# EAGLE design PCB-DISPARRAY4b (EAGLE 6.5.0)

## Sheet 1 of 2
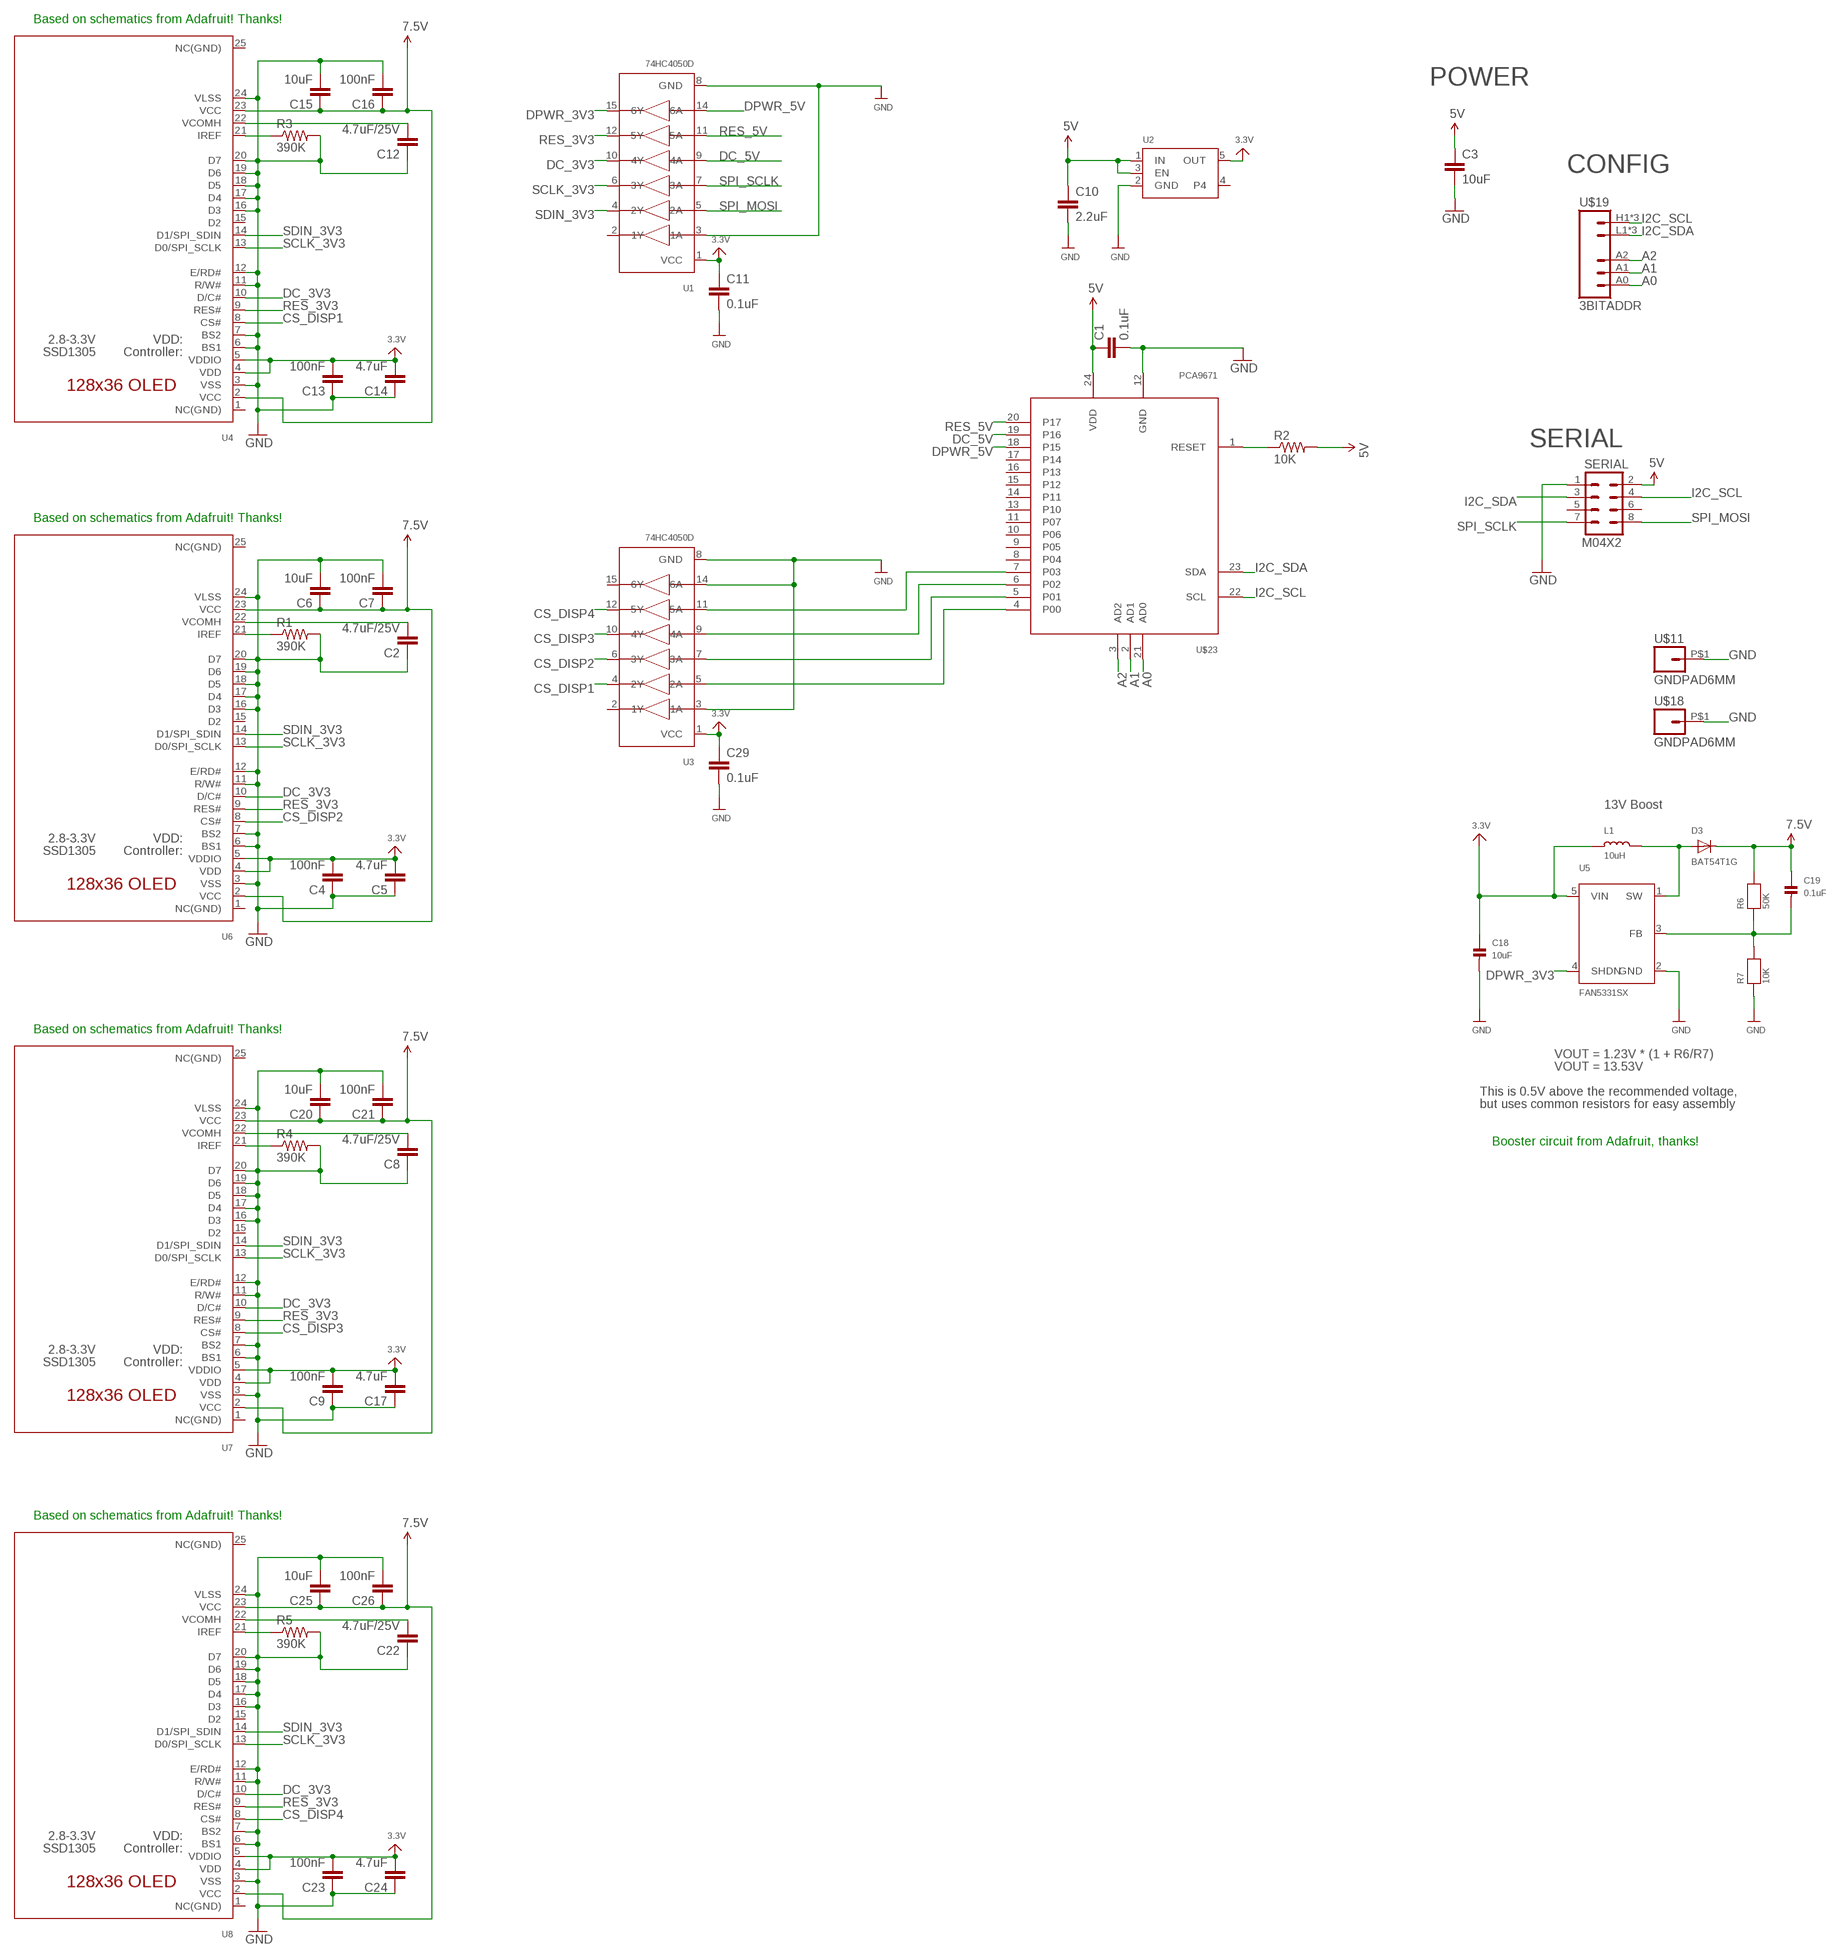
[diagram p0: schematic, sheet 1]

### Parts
C1  0.1uF  CAP0603-CAP  [0603-CAP]
C2  4.7uF/25V  CAP0805  [0805]
C3  10uF  CAP0805  [0805]
C4  100nF  CAP0603-CAP  [0603-CAP]
C5  4.7uF  CAP0603-CAP  [0603-CAP]
C6  10uF  CAP0805  [0805]
C7  100nF  CAP0603-CAP  [0603-CAP]
C8  4.7uF/25V  CAP0805  [0805]
C9  100nF  CAP0603-CAP  [0603-CAP]
C10  2.2uF  CAP0603-CAP  [0603-CAP]
C11  0.1uF  CAP0603-CAP  [0603-CAP]
C12  4.7uF/25V  CAP0805  [0805]
C13  100nF  CAP0603-CAP  [0603-CAP]
C14  4.7uF  CAP0603-CAP  [0603-CAP]
C15  10uF  CAP0805  [0805]
C16  100nF  CAP0603-CAP  [0603-CAP]
C17  4.7uF  CAP0603-CAP  [0603-CAP]
C18  10uF  CAP_CERAMIC0805  [0805]
C19  0.1uF  CAP_CERAMIC0603  [0603]
C20  10uF  CAP0805  [0805]
C21  100nF  CAP0603-CAP  [0603-CAP]
C22  4.7uF/25V  CAP0805  [0805]
C23  100nF  CAP0603-CAP  [0603-CAP]
C24  4.7uF  CAP0603-CAP  [0603-CAP]
C25  10uF  CAP0805  [0805]
C26  100nF  CAP0603-CAP  [0603-CAP]
C29  0.1uF  CAP0603-CAP  [0603-CAP]
D3  BAT54T1G  DIODESOD-123  [SOD-123]
L1  10uH  INDUCTOR  [INDUCTOR_1007]
R1  390K  RESISTOR0603-RES  [0603-RES]
R2  10K  RESISTOR0603-RES  [0603-RES]
R3  390K  RESISTOR0603-RES  [0603-RES]
R4  390K  RESISTOR0603-RES  [0603-RES]
R5  390K  RESISTOR0603-RES  [0603-RES]
R6  50K  RESISTOR0603  [0603]
R7  10K  RESISTOR0603  [0603]
SERIAL  M04X2  [2X4]
U1  74HC4050D  74HC4050DTSSOP16  [TSSOP16]
U2  VREG_SOT23-5  [SOT23-5]
U3  74HC4050D  74HC4050DTSSOP16  [TSSOP16]
U4  ER-OLED011-1TOP  [ER-OLED011-1]
U5  FAN5331SX  FAN5331  [SOT23-5]
U6  ER-OLED011-1TOP  [ER-OLED011-1]
U7  ER-OLED011-1TOP  [ER-OLED011-1]
U8  ER-OLED011-1TOP  [ER-OLED011-1]
U$11  GNDPAD6MM  [3.2MMPAD6MM]
U$18  GNDPAD6MM  [3.2MMPAD6MM]
U$19  3BITADDR  [3BITADDR]
U$23  PCA9671  [TSSOP24]

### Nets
3.3V [Power]: C4.2 C5.2 C9.2 C11.1 C13.2 C14.2 C17.2 C18.1 C23.2 C24.2 C29.1 L1.P$1 U1.1(VCC) U2.5(OUT) U3.1(VCC) U4.4(VDD) U4.5(VDDIO) U5.5(VIN) U6.4(VDD) U6.5(VDDIO) U7.4(VDD) U7.5(VDDIO) U8.4(VDD) U8.5(VDDIO)
5V [Power]: C1.1 C3.1 C10.1 R2.2 SERIAL.2 U2.1(IN) U2.3(EN) U$23.24(VDD)
7.5V [Power]: C6.1 C7.1 C15.1 C16.1 C19.1 C20.1 C21.1 C25.1 C26.1 D3.C R6.2 U4.2(VCC) U4.23(VCC) U6.2(VCC) U6.23(VCC) U7.2(VCC) U7.23(VCC) U8.2(VCC) U8.23(VCC)
A0: U$19.A0 U$23.21(AD0)
A1: U$19.A1 U$23.2(AD1)
A2: U$19.A2 U$23.3(AD2)
CS_DISP1: U3.4(2Y) U4.8(CS#)
CS_DISP2: U3.6(3Y) U6.8(CS#)
CS_DISP3: U3.10(4Y) U7.8(CS#)
CS_DISP4: U3.12(5Y) U8.8(CS#)
DC_3V3: U1.10(4Y) U4.10(D/C#) U6.10(D/C#) U7.10(D/C#) U8.10(D/C#)
DC_5V: U1.9(4A) U$23.19(P16)
DPWR_3V3: U1.15(6Y) U5.4(SHDN)
DPWR_5V [Power]: U1.14(6A) U$23.18(P15)
GND [Power]: C1.2 C2.1 C3.2 C4.1 C5.1 C6.2 C7.2 C8.1 C9.1 C10.2 C11.2 C12.1 C13.1 C14.1 C15.2 C16.2 C17.1 C18.2 C20.2 C21.2 C22.1 C23.1 C24.1 C25.2 C26.2 C29.2 R1.2 R3.2 R4.2 R5.2 R7.1 SERIAL.1 U1.3(1A) U1.8(GND) U2.2(GND) U3.3(1A) U3.8(GND) U3.14(6A) U4.3(VSS) U4.6(BS1) U4.7(BS2) U4.11(R/W#) U4.12(E/RD#) U4.16(D3) U4.17(D4) U4.18(D5) U4.19(D6) U4.20(D7) U4.24(VLSS) U5.2(GND) U6.3(VSS) U6.6(BS1) U6.7(BS2) U6.11(R/W#) U6.12(E/RD#) U6.16(D3) U6.17(D4) U6.18(D5) U6.19(D6) U6.20(D7) U6.24(VLSS) U7.3(VSS) U7.6(BS1) U7.7(BS2) U7.11(R/W#) U7.12(E/RD#) U7.16(D3) U7.17(D4) U7.18(D5) U7.19(D6) U7.20(D7) U7.24(VLSS) U8.3(VSS) U8.6(BS1) U8.7(BS2) U8.11(R/W#) U8.12(E/RD#) U8.16(D3) U8.17(D4) U8.18(D5) U8.19(D6) U8.20(D7) U8.24(VLSS) U$11.P$1 U$18.P$1 U$23.12(GND)
I2C_SCL: SERIAL.4 U$19.H1(VCC) U$19.H2(VCC) U$19.H3(VCC) U$23.22(SCL)
I2C_SDA: SERIAL.3 U$19.L1(GND) U$19.L2(GND) U$19.L3(GND) U$23.23(SDA)
N$1: R2.1 U$23.1(RESET)
N$2: R1.1 U6.21(IREF)
N$3: C2.2 U6.22(VCOMH)
N$4: R4.1 U7.21(IREF)
N$5: R3.1 U4.21(IREF)
N$6: C8.2 U7.22(VCOMH)
N$7: R5.1 U8.21(IREF)
N$8: C22.2 U8.22(VCOMH)
N$10: C12.2 U4.22(VCOMH)
N$14 [Power]: D3.A L1.P$2 U5.1(SW)
N$15: C19.2 R6.1 R7.2 U5.3(FB)
N$29: U3.5(2A) U$23.4(P00)
N$30: U3.7(3A) U$23.5(P01)
N$31: U3.9(4A) U$23.6(P02)
N$32: U3.11(5A) U$23.7(P03)
RES_3V3: U1.12(5Y) U4.9(RES#) U6.9(RES#) U7.9(RES#) U8.9(RES#)
RES_5V: U1.11(5A) U$23.20(P17)
SCLK_3V3: U1.6(3Y) U4.13(D0/SPI_SCLK) U6.13(D0/SPI_SCLK) U7.13(D0/SPI_SCLK) U8.13(D0/SPI_SCLK)
SDIN_3V3: U1.4(2Y) U4.14(D1/SPI_SDIN) U6.14(D1/SPI_SDIN) U7.14(D1/SPI_SDIN) U8.14(D1/SPI_SDIN)
SPI_MOSI: SERIAL.8 U1.5(2A)
SPI_SCLK: SERIAL.7 U1.7(3A)
Unconnected: SERIAL.5 SERIAL.6 U1.2(1Y) U2.4 U3.2(1Y) U3.15(6Y) U4.1(NC(GND)) U4.15(D2) U4.25(NC(GND)) U6.1(NC(GND)) U6.15(D2) U6.25(NC(GND)) U7.1(NC(GND)) U7.15(D2) U7.25(NC(GND)) U8.1(NC(GND)) U8.15(D2) U8.25(NC(GND)) U$23.8(P04) U$23.9(P05) U$23.10(P06) U$23.11(P07) U$23.13(P10) U$23.14(P11) U$23.15(P12) U$23.16(P13) U$23.17(P14)

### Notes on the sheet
- Based on schematics from Adafruit! Thanks!
- POWER
- CONFIG
- SERIAL
- Based on schematics from Adafruit! Thanks!
- 13V Boost
- Based on schematics from Adafruit! Thanks!
- VOUT = 1.23V * (1 + R6/R7)
- VOUT = 13.53V
- This is 0.5V above the recommended voltage,
- but uses common resistors for easy assembly
- Booster circuit from Adafruit, thanks!
- Based on schematics from Adafruit! Thanks!

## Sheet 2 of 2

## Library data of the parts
C1-C17 C20-C26 C29 = SparkFun:CAP: Capacitor
C18 C19 = microbuilder:CAP_CERAMIC: Ceramic Capacitors
D3 = microbuilder:DIODE: Diode
L1 = microbuilder:INDUCTOR: Inductors
R1-R5 = SparkFun:RESISTOR: Resistor
R6 R7 = microbuilder:RESISTOR: Resistors
SERIAL = SparkFun:M04X2
U1 U3 = SKAARHOJ:74HC4050D: 6-channel level shifter 74HC4050D - 2V-6V Supply Digikey: 74HC4050D,653-ND Mouser: 771-74HC4050D-T
U2 = microbuilder:VREG_SOT23-5: SOT23-5 Fixed Voltage Regulators To better organise some of the SOT23-5 fixed voltage regulators in this library, this new part was created. Part Current Out V Out V In V Dropout Digikey Part No. ADP121 150mA 3.3V 3.4-5.5V 0.09V @ 150mA ADP121-AUJZ33R7CT-ND ADP121 150mA 3.0V 3.1-5.5V 0.09V @ 150mA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
U4 U6-U8 = SKAARHOJ:ER-OLED011-1: UG-2864HSWEG01 OLED display Both 1.3" and 0.96" models share the same FPC tab footprint, only the screen dimensions vary.
U5 = microbuilder:FAN5331: FAN5331 - LED/OLED 20V Boost Converter Digikey: FAN5331SXCT-ND
U$11 U$18 = SKAARHOJ:GNDPAD
U$19 = SKAARHOJ:3BITADDR
U$23 = SKAARHOJ:PCA9671

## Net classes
0 default: width 0.203 mm, drill 0.305 mm, clearance 0.203 mm
1 Power: width 0.305 mm, drill 0.406 mm, clearance 0.203 mm

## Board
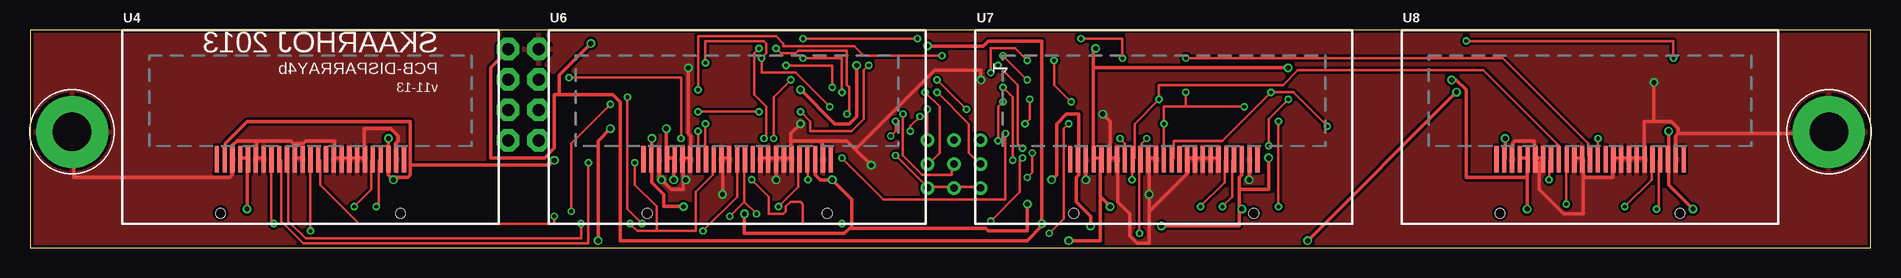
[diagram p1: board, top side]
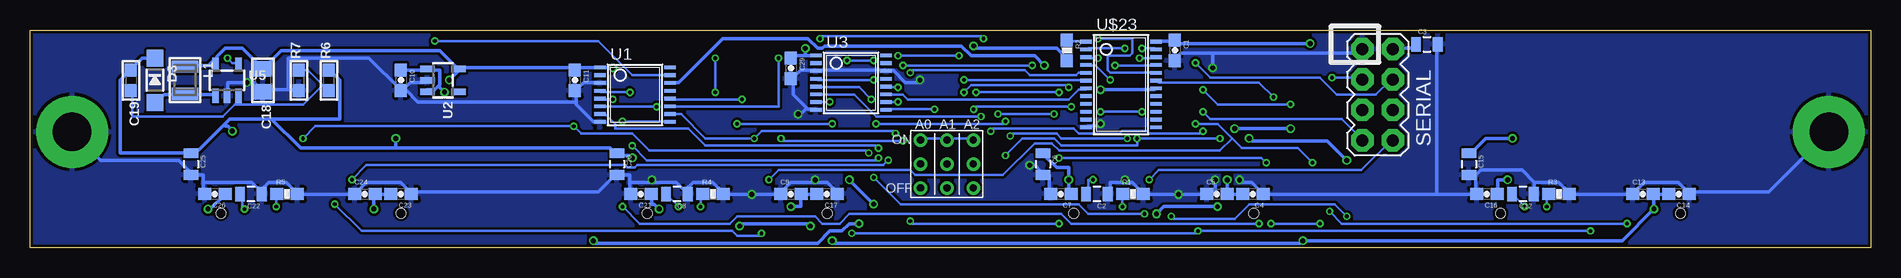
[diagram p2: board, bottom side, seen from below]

Size 153.42 x 18.2 mm. Coordinates in mm from the lower left corner, seen from the top.
Outline: 153.42,0 153.42,18.2 0,18.2 0,0 153.42,0
Copper layers (1*16): Top 0.035mm / dielectric 1.5mm / Bottom 0.035mm
Design rules "Fusion_eagle_rule_v1.1": minimum track width 6mil, minimum drill 12mil, track to track 6mil, track to pad 6mil, pad to pad 6mil, via to via 6mil, smd to smd 0mil, copper to edge 10mil, drill to drill 10mil, minimum pad ring 10mil, minimum via ring 6mil, stop-mask expansion 2mil, vias tented up to drill 100mil, thermal gap 10mil

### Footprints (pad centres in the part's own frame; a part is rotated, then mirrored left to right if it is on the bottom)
0603-CAP = smd 1.1 x 1: 1 -0.85,0; 2 0.85,0
0805 = smd 0.8 x 1.2: 1 -0.9,0; 2 0.9,0
0805' = smd 1.3 x 1.5: 1 -0.95,0; 2 0.95,0
0603 = smd 1.1 x 1: 1 -0.85,0; 2 0.85,0
SOD-123 = smd 1.4 x 1.4: A 1.85,0; C -1.85,0
INDUCTOR_1007 = smd 1.016 x 2.2: P$1 -1.127,0; P$2 1.127,0
0603-RES = smd 1.1 x 1: 1 -0.85,0; 2 0.85,0
2X4 = drill 1.016 pad 1.88 octagon: 1 -3.81,-1.27; 2 -3.81,1.27; 3 -1.27,-1.27; 4 -1.27,1.27; 5 1.27,-1.27; 6 1.27,1.27; 7 3.81,-1.27; 8 3.81,1.27
TSSOP16 = smd 0.305 x 0.991: 1 -3.575,-2.918; 2 -2.925,-2.918; 3 -2.275,-2.918; 4 -1.625,-2.918; 5 -0.975,-2.918; 6 -0.325,-2.918; 7 0.325,-2.918; 8 0.975,-2.918; 9 0.975,2.918; 10 0.325,2.918; 11 -0.325,2.918; 12 -0.975,2.918; 13 -1.625,2.918; 14 -2.275,2.918; 15 -2.925,2.918; 16 -3.575,2.918
SOT23-5 = smd 0.55 x 1.2: 1 -0.95,-1.3; 2 0,-1.3; 3 0.95,-1.3; 4 0.95,1.3; 5 -0.95,1.3
ER-OLED011-1 = smd 0.35 x 2.2: 1 -7.8,-2.7; 2 -7.15,-2.7; 3 -6.5,-2.7; 4 -5.85,-2.7; 5 -5.2,-2.7; 6 -4.55,-2.7; 7 -3.9,-2.7; 8 -3.25,-2.7; 9 -2.6,-2.7; 10 -1.95,-2.7; 11 -1.3,-2.7; 12 -0.65,-2.7; 13 0,-2.7; 14 0.65,-2.7; 15 1.3,-2.7; 16 1.95,-2.7; 17 2.6,-2.7; 18 3.25,-2.7; 19 3.9,-2.7; 20 4.55,-2.7; 21 5.2,-2.7; 22 5.85,-2.7; 23 6.5,-2.7; 24 7.15,-2.7; 25 7.8,-2.7 | hole 0.8: -7.5,-7.2; 7.5,-7.2
3.2MMPAD6MM = drill 3.2 pad 6: P$1 0,0
3BITADDR = drill 0.6: A0 -2.2,0; A1 0,0; A2 2.2,0; H1 -2.2,2; H2 0,2; H3 2.2,2; L1 -2.2,-2; L2 0,-2; L3 2.2,-2
TSSOP24 = smd 0.305 x 0.991: 1 -4.225,-2.918; 2 -3.575,-2.918; 3 -2.925,-2.918; 4 -2.275,-2.918; 5 -1.625,-2.918; 6 -0.975,-2.918; 7 -0.325,-2.918; 8 0.325,-2.918; 9 0.975,-2.918; 10 1.625,-2.918; 11 2.275,-2.918; 12 2.925,-2.918; 13 2.925,2.918; 14 2.275,2.918; 15 1.625,2.918; 16 0.975,2.918; 17 0.325,2.918; 18 -0.325,2.918; 19 -0.975,2.918; 20 -1.625,2.918; 21 -2.275,2.918; 22 -2.925,2.918; 23 -3.575,2.918; 24 -4.225,2.918

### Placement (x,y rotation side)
C1  58,16.5 270 bottom
C2  64.5,4.5 180 bottom
C3  37,17 0 bottom
C4  51.5,4.5 180 bottom
C5  54.5,4.5 0 bottom
C6  69,7 270 bottom
C7  67.5,4.5 180 bottom
C8  99.5,4.5 180 bottom
C9  90,4.5 0 bottom
C10  122.5,14 270 bottom
C11  108,14 270 bottom
C12  29,4.5 180 bottom
C13  19,4.5 0 bottom
C14  16,4.5 180 bottom
C15  33.5,7 270 bottom
C16  32,4.5 180 bottom
C17  87,4.5 180 bottom
C18  10uF  [0805']  134,14 270 bottom
C19  145,14 270 bottom
C20  104.5,7 270 bottom
C21  102.5,4.5 180 bottom
C22  135,4.5 180 bottom
C23  122.5,4.5 180 bottom
C24  125.5,4.5 0 bottom
C25  140,7 270 bottom
C26  138,4.5 180 bottom
C29  90,15 270 bottom
D3  143,14 270 bottom
L1  140.5,14 270 bottom
R1  61.5,4.5 0 bottom
R2  67,16.5 270 bottom
R3  26,4.5 0 bottom
R4  96.5,4.5 0 bottom
R5  132,4.5 0 bottom
R6  128.5,14 90 bottom
R7  131,14 90 bottom
SERIAL  41.12,12.79 270 bottom
U1  103,11.5 270 bottom
U2  119,14 270 bottom
U3  85,12.5 270 bottom
U4  23.37,10.1 0 top
U5  137,14 0 bottom
U6  58.93,10.1 0 top
U7  94.49,10.1 0 top
U8  130,10.1 0 top
U$11  149.92,9.7 0 top
U$18  3.5,9.7 0 top
U$19  77,7 0 bottom
U$23  62.5,13 270 bottom

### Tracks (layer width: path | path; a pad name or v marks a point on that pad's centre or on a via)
3.3V  (via drill 0.41)
  Top 0.305: v53.65,5.69 53.65,7.32 U6.5 53.65,7.52 53.24,7.52 U6.4 53.03,7.52 v53.03,9.96 | v18.09,3.25 18.09,7.32 U4.5 18.09,7.52 17.68,7.52 U4.4 | v48.36,9.96 47.35,8.94 v47.35,0.61 | 89.31,4.17 89.2,4.27 89.2,7.32 U7.5 89.2,7.52 88.8,7.52 U7.4 88.59,7.52 88.59,15.04 | 89.31,4.17 v90.02,3.45 | v88.8,16.66 88.59,16.46 88.59,15.04 | 124.77,5.89 124.77,7.32 U8.5 124.77,7.52 124.16,7.52 U8.4 | 124.77,5.89 v124.77,3.25 | 124.77,5.89 119.69,5.89 119.69,13.21 118.87,14.02 v118.47,14.02 | v104.85,15.04 88.59,15.04 | v86.56,0.61 89.2,0.61 89.2,4.06 89.31,4.17
  Bottom 0.305: C4.2 52.43,4.47 53.65,4.47 C5.2 53.65,4.67 v53.65,5.69 | 18.09,4.47 16.87,4.47 C14.2 | 18.09,4.47 v18.09,3.25 20.73,0.61 v47.35,0.61 47.55,0.41 86.36,0.41 v86.56,0.61 | 18.09,4.47 C13.2 | v48.36,9.96 v53.03,9.96 | C17.2 87.99,4.47 89,4.47 C9.2 89.2,4.47 89.2,3.45 v90.02,3.45 | 88.8,16.05 89.81,16.05 C29.1 | 88.8,16.05 87.99,16.05 U3.1 | v88.8,16.66 88.8,16.05 | 138.58,15.24 140.41,15.24 L1.P$1 | 138.58,15.24 137.97,15.24 U5.5 | 138.58,15.24 137.16,16.66 135.74,16.66 134.11,15.04 C18.1 133.91,15.04 132.49,16.46 119.28,16.46 117.86,15.04 U2.5 | C23.2 123.55,4.47 124.56,4.47 C24.2 124.77,4.47 v124.77,3.25 | U2.5 117.65,15.04 108.1,15.04 C11.1 107.9,15.04 106.07,15.04 U1.1 105.87,15.04 v104.85,15.04 | v118.47,14.02 117.65,14.83 U2.5
5V  (via drill 0.41)
  Top 0.305: v74.78,16.87 79.45,16.87 79.86,17.27 84.33,17.27 v84.33,2.03 84.33,1.83 83.11,0.61 49.17,0.61 49.17,12.19 48.56,12.8 44.09,12.8 | 44.09,12.8 43.69,12.8 43.69,8.33 42.88,7.52 38.41,7.52 38.41,15.04 39.83,16.46 SERIAL.2 | v46.74,17.07 44.09,14.43 44.09,12.8 | v106.48,0.61 v118.87,13.01
  Bottom 0.305: C10.1 122.33,14.83 120.5,14.83 U2.1 120.29,14.83 119.28,14.83 119.28,13.61 119.38,13.51 | 119.38,13.51 119.69,13.21 120.29,13.21 U2.3 | U$23.24 59.54,17.27 58.12,17.27 C1.1 57.91,17.27 57.71,17.07 v46.74,17.07 | v74.78,16.87 74.57,16.66 67.87,16.66 67.06,15.85 R2.2 | C3.1 38,16.87 38.2,16.66 39.83,16.66 SERIAL.2 | v118.87,13.01 119.38,13.51 | v106.48,0.61 106.27,0.41 87.78,0.41 86.77,1.42 85.75,1.42 85.14,2.03 v84.33,2.03
7.5V  (via drill 0.41)
  Top 0.305: 65.43,7.52 U6.23 65.43,7.32 65.43,6.1 65.84,5.69 v66.85,5.69 68.48,4.06 68.48,1.83 68.38,1.73 | v29.87,9.14 29.87,7.52 U4.23 29.87,7.32 29.87,6.1 v30.28,5.69 30.28,5.89 31.5,5.89 31.7,6.1 31.7,6.91 | 31.7,6.91 31.7,10.57 18.09,10.57 16.26,8.74 16.26,7.52 U4.2 | v51.82,9.14 51.82,7.52 U6.2 51.82,7.32 51.82,5.49 52.83,4.47 52.83,3.45 v54.46,3.45 | v43.69,7.32 43.28,6.91 31.7,6.91 | 68.38,1.73 67.87,1.22 59.54,1.22 v59.54,2.85 | 100.79,4.88 100.79,5.89 100.99,6.1 100.99,7.32 U7.23 100.99,7.52 | 100.79,4.88 100.79,3.45 v100.99,3.25 100.79,3.25 100.79,1.83 v94.28,1.83 | v88.39,1.83 88.39,2.64 87.17,3.86 87.17,5.89 87.38,6.1 87.38,7.32 U7.2 87.38,7.52 87.38,11.18 86.36,11.18 85.55,10.36 85.55,6.1 v85.14,5.69 | v138.58,3.25 136.55,5.28 136.55,7.32 U8.23 136.55,7.52 v136.55,9.75 | v122.94,9.14 122.94,7.52 U8.2 | 100.79,4.88 103.23,4.88 v103.23,7.52 | v83.11,3.66 83.11,1.42 79.86,1.42 79.65,1.63 68.48,1.63 68.38,1.73
  Bottom 0.305: C7.1 66.85,4.67 v66.85,5.69 66.85,6.71 67.87,6.71 68.89,7.72 C6.1 | v30.28,5.69 31.09,5.69 31.09,4.67 C16.1 | v29.87,9.14 32.11,9.14 33.33,7.92 C15.1 | v51.82,9.14 51.61,8.94 45.31,8.94 v43.69,7.32 | v59.54,2.85 58.93,3.45 v54.46,3.45 | v100.99,3.25 101.4,3.66 101.6,3.66 101.6,4.47 C21.1 | v88.39,1.83 88.59,2.03 94.08,2.03 v94.28,1.83 | v138.58,3.25 138.38,3.25 137.16,4.47 C26.1 | D3.C 143.05,15.85 144.07,15.85 144.88,15.04 C19.1 145.09,14.83 145.9,14.02 145.9,7.92 140,7.92 C25.1 139.8,7.92 139.6,7.92 137.26,10.26 | 133.3,10.77 136.75,10.77 137.26,10.26 | 133.3,10.77 127.61,10.77 127.61,14.02 128.42,14.83 R6.2 | 122.94,8.33 130.86,8.33 133.3,10.77 | 122.94,8.33 105.05,8.33 104.65,7.92 C20.1 104.44,7.72 103.43,7.72 v103.23,7.52 | 122.94,8.33 v122.94,9.14 | v136.55,9.75 136.96,10.16 137.16,10.16 137.26,10.26 | v85.14,5.69 v83.11,3.66
A0  (via drill 0.3)
  Top 0.203: v62.99,15.24 66.85,15.24 v66.85,13.41 | v75.59,13.01 78.23,10.36 78.23,7.92 79.05,7.11 U$19.A0
  Bottom 0.203: v62.99,15.24 59.74,15.24 U$23.21 | v66.85,13.41 67.06,13.61 74.98,13.61 v75.59,13.01
A1  (via drill 0.3)
  Top 0.203: v62.18,16.66 62.59,16.26 63.8,16.26 64.01,16.46 68.07,16.46 68.07,13.61 68.28,13.41 68.28,11.38 v68.07,11.18 | v72.75,11.18 72.75,7.72 74.37,6.1 76.81,6.1 76.81,6.91 U$19.A1
  Bottom 0.203: v62.18,16.66 65.23,16.66 U$23.2 | v72.75,11.18 v68.07,11.18
A2  (via drill 0.3)
  Top 0.203: v64.41,15.85 67.67,15.85 v67.67,13.01 | v74.57,13.01 75.79,11.79 75.79,7.92 74.98,7.11 U$19.A2
  Bottom 0.203: v64.41,15.85 65.23,15.85 U$23.3 | v74.57,13.01 v67.67,13.01
CS_DISP1  (via drill 0.3)
  Top 0.203: v81.08,16.05 v83.11,14.02 | v76,16.05 69.49,16.05 68.68,16.87 62.79,16.87 62.79,17.07 62.18,17.68 55.68,17.68 v55.68,13.21 | v48.36,11.99 45.11,8.74 v45.11,3.05 | v20.32,2.03 20.12,2.23 20.12,7.32 U4.8
  Bottom 0.203: v83.11,14.02 87.78,14.02 U3.4 | v76,16.05 v81.08,16.05 | v55.68,13.21 54.46,11.99 v48.36,11.99 | v45.11,3.05 44.09,2.03 v20.32,2.03
CS_DISP2  (via drill 0.3)
  Top 0.203: v74.17,10.97 73.36,10.16 v73.36,9.75 | v55.68,9.75 55.68,7.52 U6.8
  Bottom 0.203: v74.17,10.97 82.91,10.97 84.73,12.8 87.78,12.8 U3.6 | v73.36,9.75 73.15,9.96 66.45,9.96 66.04,9.55 62.59,9.55 62.38,9.75 60.35,9.75 60.15,9.55 55.88,9.55 v55.68,9.75
CS_DISP3  (via drill 0.3)
  Top 0.203: v81.08,12.19 80.67,11.79 v80.67,8.94 | v90.83,9.14 91.24,8.74 91.24,7.52 U7.8
  Bottom 0.203: v81.08,12.19 81.89,12.19 U3.10 | v80.67,8.94 90.63,8.94 v90.83,9.14
CS_DISP4  (via drill 0.3)
  Top 0.203: v81.08,13.41 81.89,12.6 v81.89,7.32 | v126.59,5.69 126.59,7.32 U8.8
  Bottom 0.203: v81.08,13.41 81.89,13.41 U3.12 | v81.89,7.32 82.3,6.91 102.82,6.91 103.02,6.71 103.63,6.71 103.83,6.91 125.37,6.91 v126.59,5.69
DC_3V3  (via drill 0.3)
  Top 0.203: v45.92,2.03 45.92,0.81 22.96,0.81 21.54,2.23 21.54,7.32 U4.10 | v49.99,2.03 50.6,1.42 52.22,1.42 | 52.22,1.42 55.47,1.42 55.47,4.67 56.9,6.1 56.9,7.32 U6.10 | v93.07,9.14 92.66,8.74 92.66,7.52 U7.10 92.46,7.32 v92.46,1.22 | v128.02,3.66 128.02,7.32 U8.10 | 52.22,1.42 52.22,3.45 50.39,5.28 v50.39,7.11 | v67.67,7.52 71.12,4.06 81.28,4.06 v81.28,9.55
  Bottom 0.203: v49.99,2.03 v45.92,2.03 | U1.10 99.97,11.18 99.16,11.18 97.13,9.14 v93.07,9.14 92.46,9.75 81.48,9.75 v81.28,9.55 | v128.02,3.66 125.78,1.42 94.89,1.42 94.49,1.02 92.66,1.02 v92.46,1.22 | v50.39,7.11 50.8,7.52 v67.67,7.52
DC_5V  (via drill 0.3)
  Top 0.203: v104.04,3.45 v104.04,10.57 | v51,2.03 49.78,3.25 v49.78,12.6
  Bottom 0.203: v104.04,10.57 100.18,10.57 U1.9 | v104.04,3.45 102.62,2.03 95.1,2.03 94.49,2.64 87.99,2.64 87.38,2.03 85.95,2.03 85.14,2.85 67.46,2.85 66.65,2.03 v51,2.03 | v49.78,12.6 51,13.82 59.33,13.82 59.54,14.02 U$23.19
DPWR_3V3  (via drill 0.3)
  Top 0.203: v119.69,17.27 136.96,17.27 v136.96,15.85
  Bottom 0.203: v119.69,17.27 106.07,17.27 103.23,14.43 100.18,14.43 U1.15 | v136.96,15.85 136.55,15.44 136.14,15.44 U5.4
DPWR_5V  (via drill 0.41)
  Top 0.305: v64.21,13.21 67.06,10.36 68.28,10.36 68.89,10.97 v68.89,15.24
  Bottom 0.305: v64.21,13.21 59.74,13.21 U$23.18 | v68.89,15.24 69.7,16.05 74.98,16.05 75.79,16.87 87.17,16.87 87.38,16.66 87.78,16.66 88.59,17.48 95.71,17.48 99.36,13.82 99.97,13.82 U1.14
GND  (via drill 0.41)
  Top 0.305: 22.15,7.52 22.55,7.52 U4.12 | 18.9,8.94 17.27,8.94 16.87,8.53 16.87,7.52 U4.3 16.87,7.32 16.87,6.1 16.66,5.89 3.66,5.89 3.66,9.55 U$18.P$1 | 18.9,7.52 18.9,8.94 | 18.9,7.52 19.3,7.52 U4.7 | 18.9,7.52 U4.6 | 22.15,7.52 22.15,8.53 22.05,8.64 | 22.05,8.64 21.74,8.94 18.9,8.94 | 22.15,7.52 U4.11 | 25.4,7.52 25.81,7.52 U4.17 26.01,7.52 26.62,7.52 | 27.84,7.52 27.43,7.52 U4.19 27.23,7.52 26.62,7.52 | 27.84,7.52 27.84,9.96 30.07,9.96 30.68,9.35 30.68,8.94 30.48,8.74 30.48,7.52 U4.24 | 27.84,7.52 U4.20 | 26.62,7.52 U4.18 | 25.4,7.52 25.4,8.94 22.96,8.94 22.76,8.74 22.15,8.74 22.05,8.64 | 25.4,7.52 U4.16 | 68.78,8.23 68.07,8.94 66.04,8.94 | 68.78,8.23 v70.1,6.91 | 66.04,8.94 66.04,7.52 U6.24 | U6.16 60.96,7.52 61.37,7.52 U6.17 61.57,7.52 62.18,7.52 | v64.21,10.36 63.4,9.55 63.4,8.94 | 63.4,7.52 63.4,8.94 | 63.4,7.52 62.99,7.52 U6.19 62.79,7.52 62.18,7.52 | 63.4,7.52 U6.20 | 62.18,7.52 U6.18 62.18,7.32 v62.18,5.69 | 63.4,8.94 66.04,8.94 | 54.46,5.69 54.46,7.32 U6.6 54.46,7.52 54.86,7.52 U6.7 55.07,7.52 55.07,9.35 54.86,9.55 v54.86,15.04 | 54.46,5.69 54.46,4.88 53.44,4.88 v52.63,5.69 52.43,5.89 52.43,7.32 U6.3 | U6.12 58.12,7.52 57.71,7.52 U6.11 57.71,7.32 v57.71,4.47 | v54.66,5.69 54.46,5.69 | U7.20 98.96,7.52 98.55,7.52 U7.19 98.35,7.52 97.74,7.52 | 97.74,7.52 97.13,7.52 U7.17 96.93,7.52 96.52,7.52 U7.16 96.52,7.32 96.52,6.3 93.27,3.05 | 97.74,7.52 U7.18 | 90.02,7.52 90.42,7.52 U7.7 90.63,7.32 90.63,3.86 91.64,2.85 91.64,1.02 92.25,0.41 93.27,0.41 93.27,3.05 | U7.12 93.67,7.52 93.27,7.52 U7.11 93.27,7.32 v93.27,4.47 93.27,3.05 | v89.41,11.18 90.02,10.57 90.02,7.52 | 90.02,7.52 U7.6 | v101.6,5.69 101.6,7.32 U7.24
  Top 0.305: v87.99,5.69 87.99,7.32 U7.3 | U8.3 123.55,7.52 123.55,8.74 123.75,8.94 125.37,8.94 125.37,7.52 U8.6 125.58,7.52 125.98,7.52 U8.7 125.98,7.32 125.78,7.11 125.78,4.88 127.81,2.85 129.44,2.85 129.44,5.89 129.54,5.99 | U8.11 128.83,7.52 129.24,7.52 U8.12 129.44,7.32 129.44,6.1 129.54,5.99 | 133.91,7.52 133.3,7.52 U8.18 133.1,7.52 132.69,7.52 U8.17 132.49,7.52 132.08,7.52 U8.16 131.88,7.32 131.88,5.89 129.64,5.89 129.54,5.99 | 133.91,7.52 134.52,7.52 | 133.91,7.52 U8.19 | 137.36,9.55 137.16,9.35 137.16,7.52 U8.24 | 137.36,9.55 137.36,9.96 136.75,10.57 135.33,10.57 | 135.33,10.57 134.52,10.57 134.52,7.52 | 134.52,7.52 U8.20 | 137.36,9.55 149.76,9.55 U$11.P$1 | 135.33,10.57 v135.33,13.82 | 68.78,8.23 75.39,14.83 79.25,14.83 v79.25,14.02
  Bottom 0.305: 54.86,16.26 42.67,16.26 42.47,16.46 SERIAL.1 | 54.86,16.26 57.51,16.26 57.91,15.85 C1.2 | C7.2 68.48,4.67 68.48,6.1 68.89,6.1 C6.2 69.09,6.3 69.7,6.91 v70.1,6.91 | v64.21,10.36 64.41,10.16 65.23,10.16 U$23.12 | 62.18,5.49 61.57,5.49 60.76,4.67 R1.2 60.55,4.47 v57.71,4.47 55.47,4.47 C5.1 55.27,4.67 54.66,4.67 v54.66,5.69 | 62.18,5.49 63.4,5.49 63.4,4.67 C2.1 | 62.18,5.49 v62.18,5.69 | v54.86,15.04 54.86,16.26 | 28.04,5.49 28.04,4.67 C12.1 | 28.04,5.49 26.01,5.49 25.2,4.67 R3.2 24.99,4.47 19.91,4.47 C13.1 19.71,4.67 18.9,5.49 16.05,5.49 15.24,4.67 C14.1 15.04,4.67 8.53,4.67 3.66,9.55 U$18.P$1 | 32.92,6.1 32.92,4.67 C16.2 32.92,4.47 36.17,4.47 | 32.92,6.1 33.33,6.1 C15.2 32.92,6.1 | 36.17,4.47 50.6,4.47 C4.1 50.8,4.67 51.61,5.49 52.43,5.49 v52.63,5.69 | 36.17,4.47 36.17,16.87 C3.2 | 28.04,5.49 29.06,6.5 32.51,6.5 32.92,6.1 | 131.88,13.21 133.91,13.21 C18.2 134.11,13.21 134.72,13.82 v135.33,13.82 136.96,13.82 136.96,12.8 U5.2 | 131.88,13.21 131.06,13.21 R7.1 | C10.2 122.33,13.21 121.72,13.82 120.5,13.82 U2.2 | 107.9,12.19 107.9,13.01 C11.2 107.9,13.21 107.29,13.82 106.07,13.82 U1.3 | 107.9,12.19 107.9,11.99 106.48,10.57 106.07,10.57 U1.8 | 107.9,12.19 121.11,12.19 122.12,13.21 C10.2 | 131.88,13.21 131.88,15.85 125.17,15.85 122.53,13.21 C10.2 | 88.7,11.68 89.81,12.8 89.81,14.02 C29.2 89.81,14.22 89.2,14.83 87.99,14.83 U3.3 87.78,14.83 82.09,14.83 U3.14 81.89,14.83 81.48,14.83 80.47,13.82 79.45,13.82 v79.25,14.02 | 88.7,11.68 88.59,11.58 87.99,11.58 U3.8 | 88.7,11.68 89.2,11.18 v89.41,11.18 | 103.43,5.49 103.43,6.1 104.44,6.1 C20.2 104.65,6.1 106.07,4.67 121.51,4.67 C23.1 121.72,4.67 122.53,5.49 125.37,5.49 126.19,4.67 C24.1 126.39,4.47 131.06,4.47 R5.2 131.27,4.67 132.08,5.49 133.5,5.49 134.11,4.88 C22.1 134.11,4.67 134.93,5.49 138.99,5.49
  Bottom 0.305: 103.43,5.49 103.43,4.67 C21.2 | 103.43,5.49 101.6,5.49 | 101.6,5.49 99.57,5.49 98.75,4.67 C8.1 98.75,4.88 98.15,5.49 96.52,5.49 95.71,4.67 R4.2 95.5,4.47 v93.27,4.47 91.03,4.47 C9.1 90.83,4.67 90.02,5.49 87.99,5.49 | 101.6,5.49 v101.6,5.69 | 87.99,5.49 86.97,5.49 86.16,4.67 C17.1 | 87.99,5.49 v87.99,5.69 | 138.99,5.49 138.99,6.1 139.8,6.1 C25.2 140,6.3 141.02,7.32 147.52,7.32 149.76,9.55 U$11.P$1 | 138.99,5.49 138.99,4.67 C26.2
  pour Top: 0,0 153,0 153,18 0,18
  pour Bottom: 0,0 153,0 153,18 0,18
I2C_SCL  (via drill 0.3)
  Top 0.203: v56.29,15.44 56.29,17.27 61.16,17.27 61.37,17.07 61.37,16.26 v60.96,15.85 60.96,14.63 63.8,14.63 v66.65,11.79 | v74.78,11.58 74.78,9.14 U$19.H3
  Bottom 0.203: U$19.H3 74.98,9.14 76.81,9.14 U$19.H2 77.01,9.14 79.05,9.14 U$19.H1 | v60.96,15.85 59.74,15.85 U$23.22 | v56.29,15.44 55.07,14.22 45.92,14.22 44.5,12.8 41.25,12.8 40.03,14.02 SERIAL.4 | v74.78,11.58 74.57,11.79 v66.65,11.79
I2C_SDA  (via drill 0.3)
  Top 0.203: v60.76,16.66 60.35,16.26 60.35,12.8 61.37,11.79 61.37,9.35 v61.16,9.14 | v72.14,7.72 74.78,5.08 U$19.L3 74.98,5.08 76.81,5.08 U$19.L2 77.01,5.08 79.05,5.08 U$19.L1 | v44.91,14.22 54.25,14.22 v54.25,9.14
  Bottom 0.203: v60.76,16.66 59.74,16.66 U$23.23 | v72.14,7.72 70.71,9.14 68.07,9.14 67.46,8.53 61.16,8.53 v61.16,9.14 v54.25,9.14 | v44.91,14.22 42.47,14.22 SERIAL.3
N$1
  Bottom 0.203: U$23.1 65.43,17.27 66.85,17.27 R2.1
N$2  (via drill 0.3)
  Top 0.203: v62.38,3.45 64.01,5.08 64.01,7.32 U6.21
  Bottom 0.203: v62.38,3.45 62.38,4.47 R1.1
N$3  (via drill 0.3)
  Top 0.203: v64.82,5.69 64.82,7.32 U6.22
  Bottom 0.203: v64.82,5.69 65.23,5.69 65.23,4.67 C2.2
N$4  (via drill 0.3)
  Top 0.203: v97.54,3.45 99.57,5.49 99.57,7.32 U7.21
  Bottom 0.203: v97.54,3.45 97.54,4.47 R4.1
N$5  (via drill 0.3)
  Top 0.203: v27.03,3.45 28.45,4.88 28.45,7.32 U4.21
  Bottom 0.203: v27.03,3.45 27.03,4.47 R3.1
N$6  (via drill 0.3)
  Top 0.203: v99.36,3.45 100.18,4.27 100.18,7.32 U7.22
  Bottom 0.203: v99.36,3.45 100.38,4.47 C8.2
N$7  (via drill 0.3)
  Top 0.203: v132.89,3.45 135.13,5.69 135.13,7.32 U8.21
  Bottom 0.203: v132.89,3.45 132.89,4.47 R5.1
N$8  (via drill 0.3)
  Top 0.203: v135.53,3.25 135.74,3.45 135.74,7.32 U8.22
  Bottom 0.203: v135.53,3.25 135.74,3.25 135.74,4.47 C22.2
N$10  (via drill 0.3)
  Top 0.203: v28.85,3.45 29.06,3.66 29.06,7.32 U4.22
  Bottom 0.203: v28.85,3.45 C12.2
N$14
  Bottom 0.305: U5.1 137.97,12.8 140.41,12.8 L1.P$2 140.61,12.8 142.24,12.8 142.85,12.19 D3.A
N$15
  Bottom 0.203: 129.03,13.61 130.25,14.83 130.86,14.83 R7.2 | 129.03,13.61 128.63,13.21 R6.1 | 136.35,11.99 136.14,12.19 136.14,12.6 U5.3 | 136.35,11.99 137.36,10.97 144.88,10.97 144.88,13.01 C19.2 | 129.03,13.61 130.66,11.99 136.35,11.99
N$29  (via drill 0.3)
  Top 0.203: v63.4,14.02 61.98,12.6 v61.98,9.14 | v71.73,9.35 72.14,9.75 v72.14,10.57 | v82.91,10.36 83.31,10.77 v83.31,12.39
  Bottom 0.203: v63.4,14.02 64.62,15.24 65.23,15.24 U$23.4 | v61.98,9.14 67.46,9.14 67.87,9.55 71.53,9.55 v71.73,9.35 | v72.14,10.57 72.34,10.36 v82.91,10.36 | v83.31,12.39 84.33,13.41 87.78,13.41 U3.5
N$30  (via drill 0.3)
  Top 0.203: v86.77,12.19 85.34,13.61 v85.34,15.65 | v83.11,15.65 82.09,16.66 80.06,16.66 v80.06,14.63
  Bottom 0.203: v86.77,12.19 87.78,12.19 U3.7 | v83.11,15.65 v85.34,15.65 | v80.06,14.63 79.86,14.83 70.51,14.83 70.1,14.43 66.24,14.43 66.04,14.63 U$23.5
N$31  (via drill 0.3)
  Top 0.203: v75.59,14.02 v78.03,11.58
  Bottom 0.203: v78.03,11.58 81.89,11.58 U3.9 | v75.59,14.02 65.43,14.02 U$23.6
N$32
  Bottom 0.203: U$23.7 65.43,13.21 66.04,13.21 66.85,12.39 80.26,12.39 80.67,12.8 81.89,12.8 U3.11
RES_3V3  (via drill 0.3)
  Top 0.203: U8.9 127.41,7.52 127.41,8.53 121.11,14.83 105.66,14.83 104.44,13.61 94.08,13.61 v94.08,12.39 92.05,10.36 92.05,7.52 U7.9 91.85,7.32 v91.85,5.69 | v46.53,7.11 46.53,0.41 22.76,0.41 20.93,2.23 20.93,7.32 U4.9 | v56.29,10.36 56.29,7.52 U6.9
  Bottom 0.203: v94.08,12.39 99.97,12.39 U1.12 | v46.53,7.11 47.75,8.33 52.43,8.33 53.24,9.14 | 53.24,9.14 54.46,10.36 v56.29,10.36 | v91.85,5.69 91.03,6.5 80.06,6.5 79.65,6.1 72.34,6.1 69.7,8.74 68.28,8.74 67.67,8.13 54.25,8.13 53.24,9.14
RES_5V  (via drill 0.3)
  Top 0.203: v73.97,17.48 v64.41,17.48 | v87.58,17.48 91.03,17.48 v91.03,15.85
  Bottom 0.203: v64.41,17.48 61.57,17.48 61.57,16.26 61.77,16.05 63.6,16.05 63.6,14.83 63.4,14.63 59.74,14.63 U$23.20 | v73.97,17.48 74.17,17.68 87.38,17.68 v87.58,17.48 | v91.03,15.85 91.03,11.79 99.97,11.79 U1.11
SCLK_3V3  (via drill 0.3)
  Top 0.203: v23.37,1.42 U4.13 | v56.08,1.42 58.93,4.27 U6.13 | 96.32,11.79 94.49,11.79 v94.49,10.36 U7.13 | 96.32,11.79 v101.19,11.79 | v96.32,15.85 122.73,15.85 129.84,8.74 129.84,7.72 130.05,7.52 U8.13 | 96.32,11.79 v96.32,13.01 | v84.94,1.22 86.16,2.44 86.16,9.96 v86.56,10.36
  Bottom 0.203: v23.37,1.42 v56.08,1.42 56.29,1.22 v84.94,1.22 | v101.19,11.79 105.87,11.79 U1.6 | v96.32,13.01 v96.32,15.85 | v94.49,10.36 v86.56,10.36
SDIN_3V3  (via drill 0.3)
  Top 0.203: v43.69,2.64 43.69,2.03 27.43,2.03 24.18,5.28 24.18,7.32 U4.14 | 59.54,3.86 v58.32,2.64 | 59.54,3.86 59.54,7.32 U6.14 | U7.14 95.3,7.52 95.3,8.94 99.36,8.94 v103.43,13.01 105.26,13.01 v108.1,10.16 | v130.66,9.14 130.66,7.52 U8.14 | v60.55,2.85 59.54,3.86 | v83.11,5.89 83.52,6.3 v83.52,7.92
  Bottom 0.203: v43.69,2.64 44.7,3.66 51.82,3.66 53.03,2.44 58.12,2.44 v58.32,2.64 | v103.43,13.01 105.87,13.01 U1.4 | v130.66,9.14 129.64,10.16 v108.1,10.16 107.49,9.55 103.23,9.55 101.8,8.13 83.72,8.13 v83.52,7.92 | v60.55,2.85 65.23,2.85 66.04,3.66 80.87,3.66 v83.11,5.89
SPI_MOSI  (via drill 0.3)
  Top 0.203: v104.85,12.39 103.23,10.77 v103.23,8.53 | v82.7,7.52 82.5,7.32 82.5,4.67 v80.06,2.23 | v67.67,2.03 64.41,2.03 64.41,3.66 64.21,3.86 63.4,3.86 62.99,3.45 62.99,3.05 62.79,2.85 61.57,2.85 61.57,4.27 v60.15,5.69
  Bottom 0.203: v104.85,12.39 105.87,12.39 U1.5 | v103.23,8.53 102.01,7.32 82.91,7.32 v82.7,7.52 | v80.06,2.23 79.86,2.03 v67.67,2.03 | v60.15,5.69 59.33,6.5 42.47,6.5 40.03,8.94 SERIAL.8
SPI_SCLK  (via drill 0.3)
  Top 0.203: v82.7,8.33 82.3,8.74 82.3,13.61 v80.67,15.24 | v69.9,15.24 69.49,14.83 69.49,10.77 68.48,9.75 65.02,9.75 65.02,10.57 v64.21,11.38 | v55.68,11.38 v60.76,11.38
  Bottom 0.203: v82.7,8.33 82.91,8.53 97.13,8.53 98.55,9.96 104.65,9.96 104.65,10.36 105.46,11.18 105.87,11.18 U1.7 | v69.9,15.24 v80.67,15.24 | v60.76,11.38 v64.21,11.38 | v55.68,11.38 55.07,10.77 44.09,10.77 42.47,9.14 SERIAL.7

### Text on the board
_tsilk: SKAARHOJ 2013 | 1 | PCB-DISPARRAY4b | v11-13

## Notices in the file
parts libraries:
SparkFun: Licensing: CC v3.0 Share-Alike You are welcome to use this library for commercial purposes.
